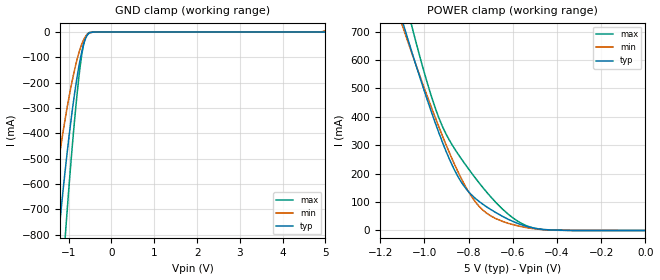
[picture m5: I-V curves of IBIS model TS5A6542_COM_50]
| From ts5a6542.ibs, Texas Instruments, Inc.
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[Model]   TS5A6542_COM_50
Model_type  Terminator
| variable   typ   min   max
C_comp   110.36pF   83.65pF   130.90pF
| C_tri-state   110.36pF   83.65pF   130.90pF
[Temperature Range]   40   100   -40
| Ambient temperature   25   85   -40
[Voltage range]   5   4.5   5.5
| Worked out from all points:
|   GND clamp passes 1 mA (typ) near -0.44 V on its own axis
|   POWER clamp passes 1 mA (typ) near -0.39 V on its own axis
[GND Clamp]
| TS5A6542_COM_50
|   Voltage   I(typ)   I(min)   I(max)
-5V       -10.62A    -7.956A    -13.58A
-1.485V   -1.28A     -830.1mA   -1.872A
-1.435V   -1.179A    -761.7mA   -1.73A
-1.255V   -837.4mA   -533.3mA   -1.24A
-1.215V   -766.5mA   -486.6mA   -1.137A
-1.095V   -566.5mA   -356.1mA   -840.8mA
-1.06V    -512.1mA   -320.9mA   -759.1mA
-885mV    -270.2mA   -166.3mA   -389.8mA
-735mV    -111.1mA   -67.43mA   -139.6mA
-635mV    -39.72mA   -25.43mA   -36.94mA
-530mV    -6.241mA   -5.165mA   -3.172mA
5V        10.27nA    5.755mA    5.34nA
[POWER Clamp]
| TS5A6542_COM_50
|   Voltage   I(typ)   I(min)   I(max)
-5V       14.71A     13.05A     17.38A
-1.115V   777mA      756.5mA    900.3mA
-1.08V    686.9mA    676.5mA    790mA
-1.05V    611.5mA    609.3mA    698.5mA
-955mV    388mA      406.2mA    440.7mA
-920mV    314.2mA    336.4mA    369.2mA
-875mV    230.9mA    252.6mA    302mA
-790mV    127.8mA    123.5mA    205.9mA
-720mV    84.01mA    61.8mA     136.6mA
-620mV    39.2mA     25.13mA    56.8mA
-510mV    9.246mA    6.726mA    9.298mA
-84.45fV  10.27nA    30.72nA    5.93nA
